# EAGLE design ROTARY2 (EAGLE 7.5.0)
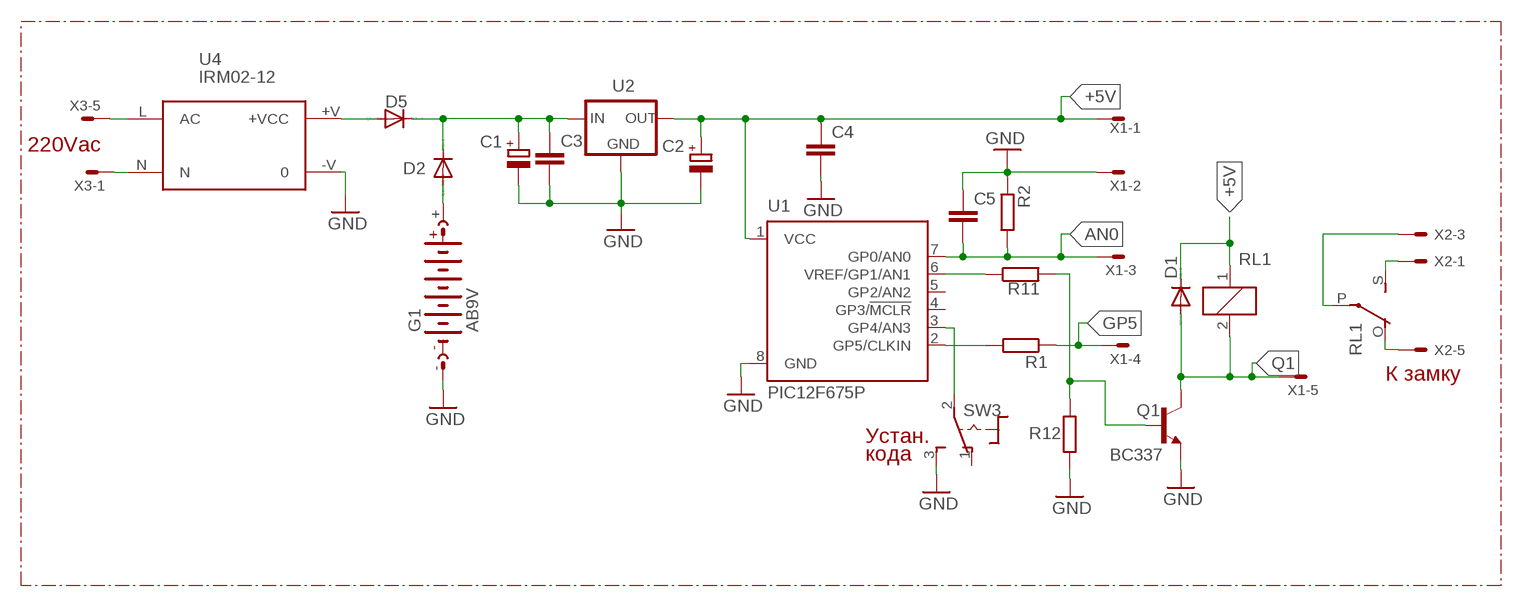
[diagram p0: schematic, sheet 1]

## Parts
C1  CPOL-EUE5-8.5  [E5-8,5]
C2  CPOL-EUE5-8.5  [E5-8,5]
C3  C-EUC1206  [C1206]
C4  C-EUC1206  [C1206]
C5  C-EUC1206  [C1206]
D1  1N4004  [DO41-10]
D2  1N4004  [DO41-10]
D5  1N4004  [DO41-10]
G1  AB9V  [AB9V]
Q1  BC337  [TO92]
R1  R-EU_M1206  [M1206]
R2  R-EU_M1206  [M1206]
R11  R-EU_M1206  [M1206]
R12  R-EU_M1206  [M1206]
RL1  G5LE  [G5LE]
SW3  8MS9P1  [8MS9]
U1  PIC12F675P  [DIL8]
U2  78XXL  [78XXL]
U4  IRM02-12  IRM02  [IRM02]
X1  22-23-2051  [22-23-2051]
X2  22-23-2051  [22-23-2051]
X3  22-23-2051  [22-23-2051]

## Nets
+5V: C2.+ C4.1 D1.C RL1.1 U1.1(VCC) U2.OUT X1.1
AN0: C5.2 R2.2 U1.7(GP0/AN0) X1.3
GND: C1.- C2.- C3.2 C4.2 C5.1 G1.- Q1.1(E) R2.1 R12.1 SW3.3(S) U1.8(GND) U2.GND U4.-V X1.2
GP5: R1.1 X1.4
N$1: R1.2 U1.2(GP5/CLKIN)
N$2: RL1.S(2:S) X2.1
N$3: SW3.2(P) U1.3(GP4/AN3)
N$4: RL1.P(2:P) X2.3
N$5: R11.1 U1.6(VREF/GP1/AN1)
N$6: Q1.2(B) R11.2 R12.2
N$7: RL1.O(2:O) X2.5
N$8: C1.+ C3.1 D2.C D5.C U2.IN
N$9: U4.N X3.1
N$10: U4.L(AC) X3.5
N$11: D5.A U4.+V(+VCC)
N$12: D2.A G1.+
Q1: D1.A Q1.3(C) RL1.2 X1.5
Unconnected: SW3.1(O) U1.4(GP3/!MCLR) U1.5(GP2/AN2) X2.2 X2.4 X3.2 X3.3 X3.4

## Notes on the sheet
- 220Vac
- К замку
- Устан.
- кода

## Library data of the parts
C1 C2 = rcl:CPOL-EU: POLARIZED CAPACITOR, European symbol
C3-C5 = rcl:C-EU: CAPACITOR, European symbol
D1 D2 D5 = diode:1N4004: DIODE
G1 = battery:AB9V: 9-V BATTERY CLIP
Q1 = transistor:BC337: NPN TRANSISTOR
R1 R2 R11 R12 = rcl:R-EU_: RESISTOR, European symbol
RL1 = relay:G5LE: RELAY 1 x switch, 10 A/120 V AC, 8 A/30 V DC, Omron; OC_FARNELL: unknown; OC_NEWARK: unknown
SW3 = switch:8MS9P1
U1 = microchip:PIC12F675: 8-Pin FLASH-Based 8-Bit CMOS Microcontroller Precision Internal 4 MHz oscillator factory calibrated to ±1% Low Power Features: Standby Current: - 1 nA @ 2.0V, typical Operating Current: - 8.5&micro;A @ 32 kHz, 2.0V, typical - 100&micro;A @ 1 MHz, 2.0V, typical Watchdog Timer Current: - 300 nA @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; MF: MICROCHIP; MPN: PIC12F675-E/P; OC_FARNELL: 9759018; OC_NEWARK: 92C4340
U2 = v-reg:78XXL: VOLTAGE REGULATOR
U4 = acdc:IRM02: 2W Single Output ACDC converter
X1-X3 = con-molex:22-23-2051: .100" (2.54mm) Center Header - 5 Pin; MF: MOLEX; MPN: 22-23-2051; OC_FARNELL: 1462952; OC_NEWARK: 38C9178

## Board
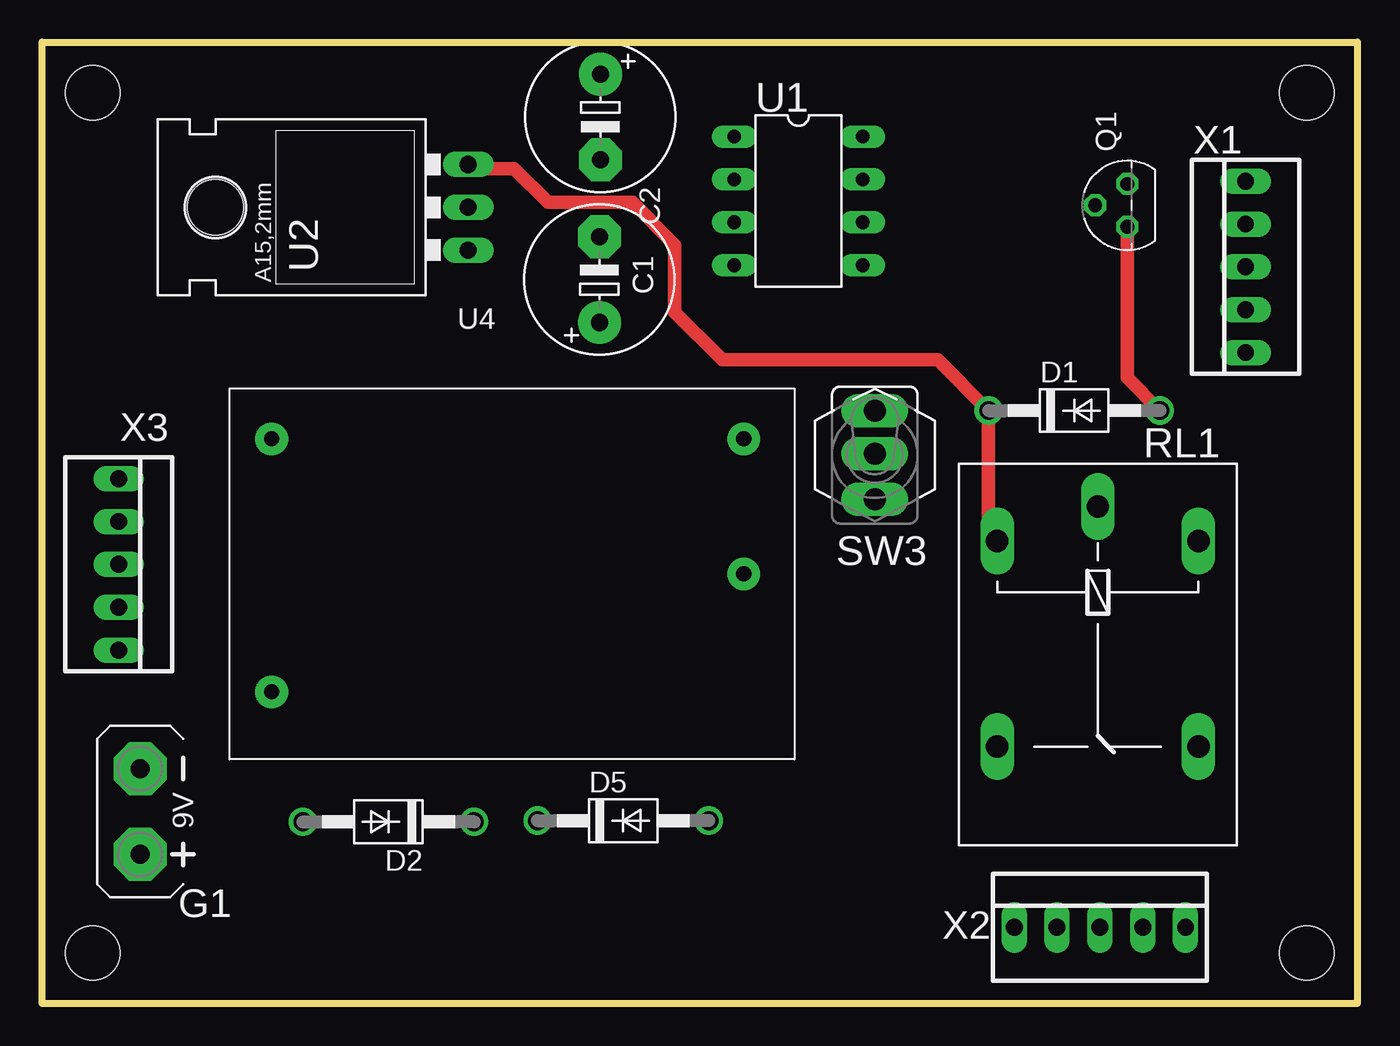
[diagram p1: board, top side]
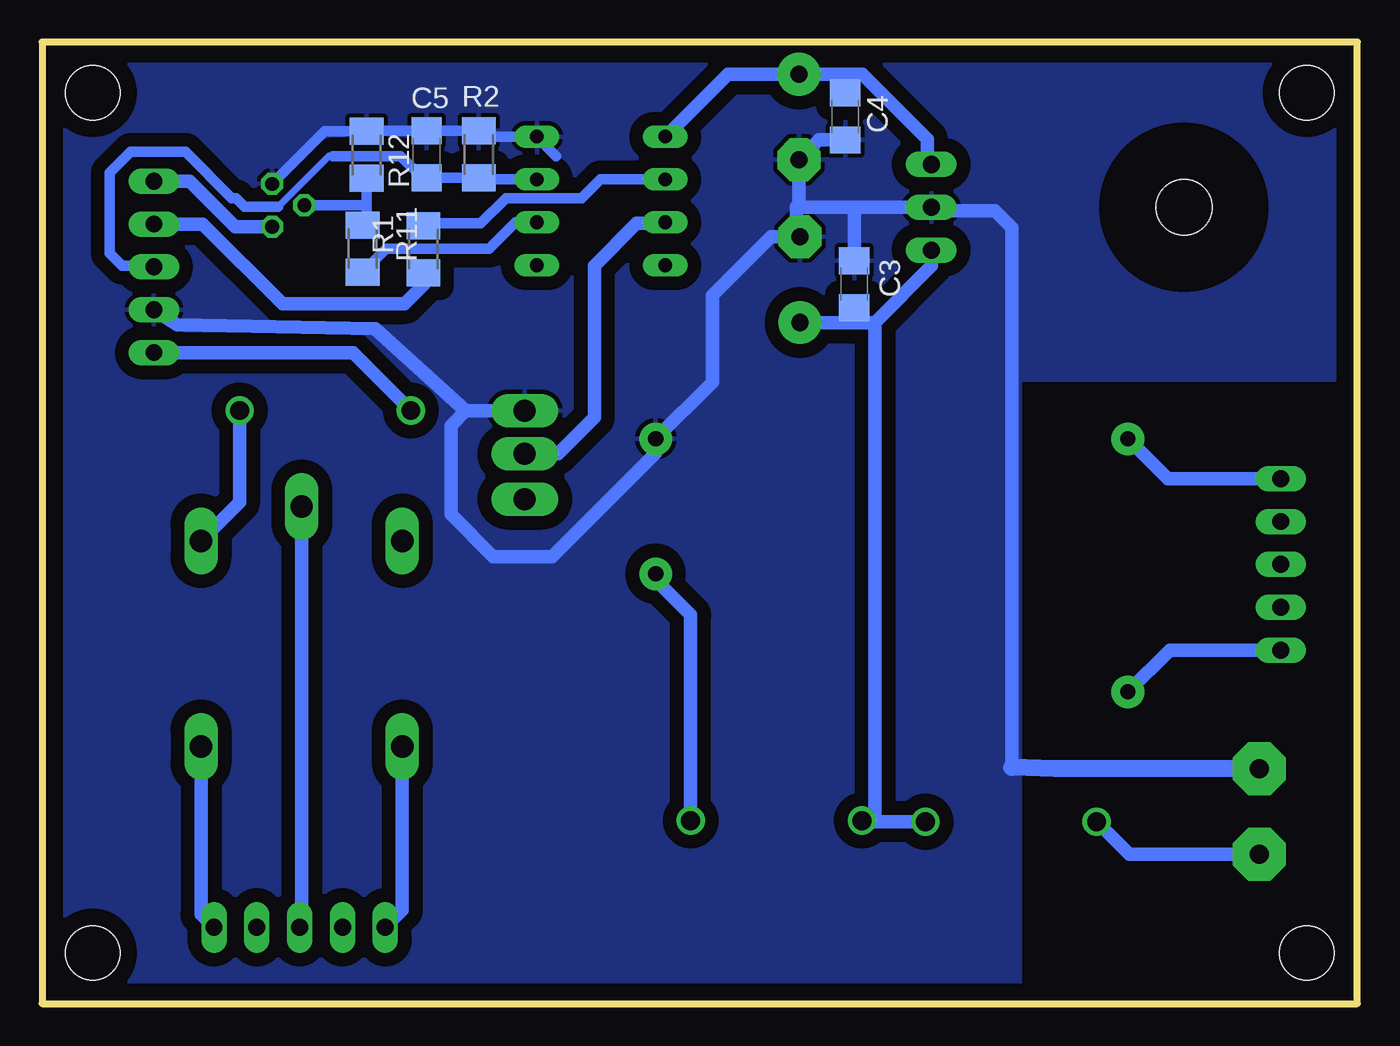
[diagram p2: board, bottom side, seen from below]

Size 78 x 57 mm. Coordinates in mm from the lower left corner, seen from the top.
Outline: 0,0 0,57 78,57 78,0 0,0
Copper layers (1*16): Top 0.035mm / dielectric 1.5mm / Bottom 0.035mm
Design rules "default": minimum track width 10mil, minimum drill 24mil, track to track 8mil, track to pad 8mil, pad to pad 8mil, via to via 8mil, smd to smd 8mil, copper to edge 40mil, drill to drill 8mil, minimum pad ring 10mil, minimum via ring 8mil, stop-mask expansion 4mil, vias tented up to drill 0mil, thermal gap 10mil
Holes 3.2 mm at 3,3 3,54 75,54 75,3

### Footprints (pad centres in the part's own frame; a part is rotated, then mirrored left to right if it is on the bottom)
E5-8,5 = drill 1.016 pad 2.54: + -2.54,0 | drill 1.016 pad 2.54 octagon: - 2.54,0
C1206 = smd 1.6 x 1.8: 1 -1.4,0; 2 1.4,0
DO41-10 = drill 1.118: A 5.08,0; C -5.08,0
AB9V = drill 1.118 pad 3.15 octagon: + 0,2.54; - 0,-2.54
TO92 = drill 0.813 octagon: 1 1.27,0; 2 0,1.905; 3 -1.27,0
M1206 = smd 1.6 x 2: 1 -1.4,0; 2 1.4,0
G5LE = drill 1.321 long: 1 -7.493,-5.969; 2 -7.493,5.969; O 4.699,5.969; P -9.525,0; S 4.699,-5.969
8MS9 = drill 1.295 pad 2 long: 1 -3,5.346 | drill 1.3 pad 2 long: 2 -3,2.654; 3 -3,0.114
DIL8 = drill 0.813 long: 1 -3.81,-3.81; 2 -1.27,-3.81; 3 1.27,-3.81; 4 3.81,-3.81; 5 3.81,3.81; 6 1.27,3.81; 7 -1.27,3.81; 8 -3.81,3.81
78XXL = drill 1.016 long: GND 0,-3.81; IN -2.54,-3.81; OUT 2.54,-3.81 | hole 3.302: 0,11.176
IRM02 = drill 0.9 pad 1.93: +V 30.5,-11; -V 30.5,-3; L 2.5,-18; N 2.5,-3
22-23-2051 = drill 1 long: 1 -5.08,0; 2 -2.54,0; 3 0,0; 4 2.54,0; 5 5.08,0

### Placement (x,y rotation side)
C1  33.05,42.92 90 top
C2  33.11,52.56 270 top
C3  29.83,42.65 90 bottom
C4  30.37,52.6 270 bottom
C5  55.2,50.35 270 bottom
D1  61.21,35.16 0 top
D2  20.54,10.78 180 top
D5  34.46,10.85 0 top
G1  5.81,11.39 180 top
Q1  64.36,47.33 90 top
R1  55.39,44.73 90 bottom
R2  52.11,50.35 270 bottom
R11  58.99,44.76 90 bottom
R12  58.76,50.32 270 bottom
RL1  62.61,19.94 270 top
SW3  46.38,35.25 180 top
U1  44.85,47.59 270 top
U2  21.46,47.21 90 top
U4  11.11,36.48 0 top
X1  71.37,43.68 90 top
X2  62.73,4.52 0 top
X3  4.54,26.04 270 top

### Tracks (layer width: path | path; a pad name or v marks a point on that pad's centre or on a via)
+5V
  Top 0.813: RL1.1 56.13,27.94 D1.C 53.13,38.16 40.34,38.16 37.5,41 37.5,45 35,47.5 30,47.5 28,49.5 25.52,49.5 U2.OUT
  Bottom 0.813: 30.25,55.1 C2.+ 37.34,55.1 U1.1 | 30.25,55.1 29.35,55.1 25.5,51.25 25.5,49.98 U2.OUT | C4.1 30.37,54.98 30.25,55.1 | X1.1 59.57,38.6 D1.C
AN0
  Bottom 0.406: 60.75,50.25 61,50.25 64,47.25
  Bottom 0.61: 51.8,48.86 R2.2 | U1.7 52.02,48.86 R2.2 | R2.2 C5.2 55.45,48.95 56.75,50.25 60.75,50.25 | 64,47.25 66,47.25 66.5,47.75 66.75,47.75 69.5,50.5 72.75,50.5 74,49.25 74,44.5 73.25,43.75 71.44,43.75 X1.3
GND
  Bottom 0.61: C2.- 33.77,50.02 34,50.25 | 47.51,50.25 U1.8 51.76,51.4 R2.1 C5.1 58.73,51.75 R12.1 | 58.27,52 R12.1 | R12.1 61.24,51.72 Q1.1
  Bottom 0.813: 30,47.21 U2.GND 25.06,47 21.5,47 20.5,46 20.5,14 | 30,47.21 33.21,47.21 33.25,47.25 | 33.25,47.25 33.25,45.76 | 33.25,47.25 33.11,47.39 C2.- 31.93,51.2 C4.2 | C3.2 29.83,47.04 30,47.21 | C1.- 34.79,45.46 38.25,42 38.25,36.84 U4.-V 41.61,32.64 47.75,26.5 51.25,26.5 53.75,29 53.75,34.27 52.89,35.14 | 72.39,41.14 X1.2 69.98,40.25 58.25,40 52.89,35.14 | SW3.3 52.89,35.14
  Bottom 1.016: G1.- 17.93,13.93 20.5,14
  pour Bottom (isolate 0.813): 0.5,56.5 0.5,37 20,37 20,34.5 20,1 77.5,1 77.5,56.5
GP5
  Bottom 0.813: R1.1 55.39,42.61 56.25,41.75 56.5,41.5 63.75,41.5 68.47,46.22 X1.4
N$1
  Bottom 0.61: U1.2 44.89,48.86 46,47.75 50.5,47.75 52,46.25 55.27,46.25 R1.2
N$2
  Bottom 0.813: RL1.S 56.64,5.53 X2.1
N$3
  Bottom 0.813: SW3.2 47.4,32.6 45.25,34.75 45.25,43.75 42.75,46.25 41.11,46.25 U1.3
N$4
  Bottom 0.813: RL1.P 62.61,4.64 X2.3
N$5
  Bottom 0.61: U1.6 49.93,46.32 51.5,44.75 57.6,44.75 R11.1
N$6
  Bottom 0.61: R12.2 58.76,47.25 | 58.76,47.25 58.76,46.39 R11.2 | Q1.2 58.84,47.33 58.76,47.25
N$7
  Bottom 0.813: RL1.O 68.58,5.29 X2.5
N$8
  Bottom 0.813: C1.+ 29.75,40.38 | 29.75,40.38 28.62,40.38 | 28.62,40.38 25.25,43.75 25.25,44.65 U2.IN | C3.1 29.83,40.46 29.75,40.38 | D2.C 28.75,10.78 | 28.75,10.78 29.31,10.78 D5.C | 28.62,40.38 28.62,10.91 28.75,10.78
N$9
  Bottom 0.813: X3.1 11.25,31.12 U4.N
N$10
  Bottom 0.813: X3.5 11.13,20.96 U4.L
N$11
  Bottom 0.813: D5.A 39.54,23.04 42,25.5 41.63,25.5 U4.+V
N$12
  Bottom 0.813: G1.+ 13.53,8.85 D2.A
Q1
  Top 0.813: Q1.3 64.36,37.09 D1.A
  Bottom 0.813: D1.A 66.29,29.72 RL1.2 | Q1.3 66.56,46.06 69.25,48.75 X1.5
